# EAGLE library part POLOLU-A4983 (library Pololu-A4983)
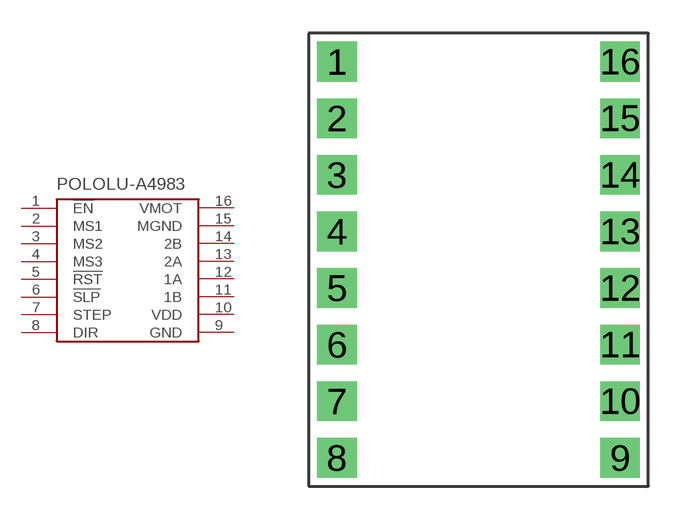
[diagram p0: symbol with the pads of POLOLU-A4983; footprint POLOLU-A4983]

Designator prefix -

## POLOLU-A4983POLOLU-A4983  [POLOLU-A4983]
1  !EN
2  MS1
3  MS2
4  MS3
5  !RST
6  !SLP
7  STEP
8  DIR
9  GND
10  VDD
11  1B
12  1A
13  2A
14  2B
15  MGND
16  VMOT

## Footprint POLOLU-A4983 (pad centres in mm)
drill 1 pad 1.778 square: 1 -6.35,8.89; 2 -6.35,6.35; 3 -6.35,3.81; 4 -6.35,1.27; 5 -6.35,-1.27; 6 -6.35,-3.81; 7 -6.35,-6.35; 8 -6.35,-8.89; 9 6.35,-8.89; 10 6.35,-6.35; 11 6.35,-3.81; 12 6.35,-1.27; 13 6.35,1.27; 14 6.35,3.81; 15 6.35,6.35; 16 6.35,8.89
